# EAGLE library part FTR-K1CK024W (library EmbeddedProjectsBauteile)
Leistungsrelais
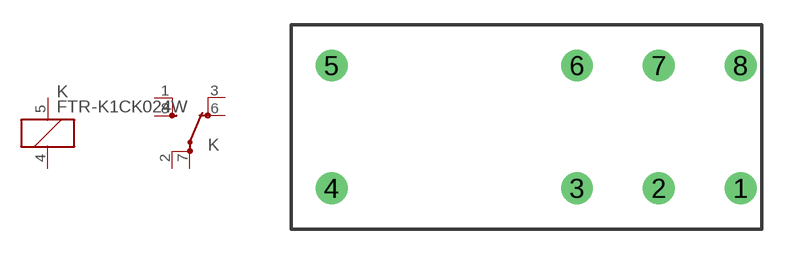
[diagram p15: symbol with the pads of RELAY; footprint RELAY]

Designator prefix K; gates G$1=K G$2=UX-2

## FTR-K1CK024W (EP: 400200)  [RELAY]
1  G$2:SBNO  pas
2  G$2:PBCOM  pas
3  G$2:OBNC  pas
4  G$1:2  pas
5  G$1:1  pas
6  G$2:OANC  pas
7  G$2:PACOM  pas
8  G$2:SANO  pas

## Footprint RELAY (pad centres in mm)
drill 1.3 pad 1.93: 1 12.5,-3.75; 2 7.5,-3.75; 3 2.5,-3.75; 4 -12.5,-3.75; 5 -12.5,3.75; 6 2.5,3.75; 7 7.5,3.75; 8 12.5,3.75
